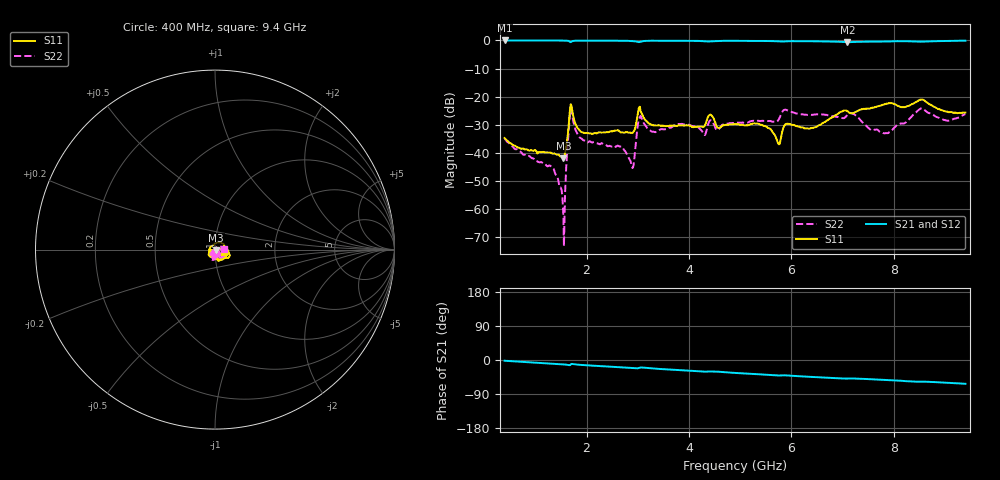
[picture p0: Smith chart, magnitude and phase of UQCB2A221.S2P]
!  Part Number  UQCB7A221	Mounting Orientation: Vertical
!  Description: RF capacitors
!  Application: Coupling, Bypass, Tuning, DC Block
!  Filters, Matching
# GHZ S DB R 50
! Freq  |S11|  S11 Ph  |S21|  S21 Ph  |S12|  S12 Ph  |S22|  S22 Ph
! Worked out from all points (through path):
!   801 points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, 400 MHz to 9.4 GHz, reference 50 ohm
!   highest |S21| = -0.02 dB at 400 MHz (marker M1); lowest = -0.6 dB at 7.094 GHz (marker M2)
!   group delay of S21, straight-line fit = 18.5 ps
!   lowest |S11| = -41.9 dB at 1.548 GHz (marker M3), VSWR 1.02, Z = 50.7 - j0.413 ohm
!   |S11| at or under -10 dB: start of sweep to end of sweep
!   |S22| runs from -73.1 to -24.1 dB; largest |S21 - S12| = 0.0056
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0.4  -34.65 -85.5  -0.02 -1.9  -0.01 -1.9  -34.85 -87.2
1.323  -40.12 -66.8  -0.05 -9.5  -0.03 -9.6  -45.07 -106.5
1.548  -41.88 -30.4  -0.07 -11.6  -0.05 -11.6  -62.46 -105.8
1.593  -38.72 -0.9  -0.09 -12.1  -0.07 -12.2  -48.73 80.8
1.649  -30.76 14.5  -0.20 -13.3  -0.18 -13.4  -33.08 45.4
1.694  -22.63 -35.2  -0.62 -11.5  -0.60 -11.6  -24.23 -26.7
1.908  -32.61 -87.0  -0.08 -13.1  -0.06 -13.2  -34.94 -110.0
2.661  -32.60 -87.9  -0.13 -19.1  -0.11 -19.2  -37.66 -140.8
2.886  -32.90 -67.9  -0.21 -21.3  -0.19 -21.4  -44.67 150.9
3.044  -23.58 -73.5  -0.53 -20.1  -0.51 -20.2  -27.47 -58.3
3.404  -30.09 -111.3  -0.11 -23.4  -0.10 -23.5  -31.94 -106.6
4.293  -30.68 -115.9  -0.28 -30.6  -0.27 -30.8  -33.47 -133.0
4.416  -26.37 -129.9  -0.34 -30.3  -0.33 -30.5  -28.38 -124.6
4.9  -29.76 -140.2  -0.15 -34.1  -0.14 -34.3  -29.35 -122.3
5.474  -30.40 -162.4  -0.21 -38.6  -0.21 -38.8  -28.57 -113.1
5.744  -36.54 -164.5  -0.34 -40.8  -0.34 -41.0  -28.34 -93.0
5.913  -29.59 -161.6  -0.32 -40.7  -0.32 -40.9  -24.77 -106.7
6.408  -31.07 119.8  -0.31 -44.8  -0.31 -45.0  -26.46 -107.0
7.094  -25.09 22.2  -0.62 -49.0  -0.63 -49.2  -26.52 -93.2
7.904  -22.31 -9.8  -0.38 -52.8  -0.40 -53.0  -32.71 -51.5
8.534  -21.01 -24.0  -0.45 -57.3  -0.48 -57.5  -24.15 -32.1
9.4  -25.63 -16.0  -0.10 -62.8  -0.12 -63.0  -26.17 2.6
